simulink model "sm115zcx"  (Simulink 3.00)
settings: Solver=ode45  SolverMode=SingleTasking  StartTime=0.0  StopTime=2.0  RelTol=1e-3  AbsTol=1e-6

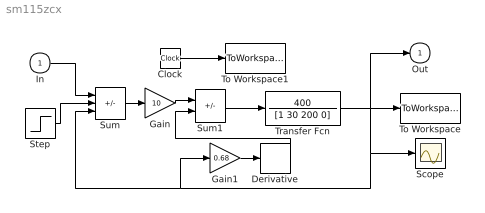
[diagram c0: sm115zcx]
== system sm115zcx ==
  In : Inport  Port=1  PortWidth=-1  SampleTime=-1  DataType=auto
  Clock : Clock
  Derivative : Derivative
  Gain : Gain  Gain=10  SaturateOnIntegerOverflow=on
  Gain1 : Gain  Gain=0.68  SaturateOnIntegerOverflow=on
  Scope : Scope
  Step : Step  Time=0  Before=0  After=1  SampleTime=0
  Sum : Sum  Inputs=++-  SaturateOnIntegerOverflow=on
  Sum1 : Sum  Inputs=+-  SaturateOnIntegerOverflow=on
  To Workspace : ToWorkspace  VariableName=y3  SampleTime=-1  SaveFormat=Matrix
  To Workspace1 : ToWorkspace  VariableName=t3  SampleTime=-1  SaveFormat=Matrix
  Transfer Fcn : TransferFcn  Numerator=400  Denominator=[1 30 200 0]
  Out : Outport  Port=1  InitialOutput=0
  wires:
  Clock/1 -> To Workspace1/1
  Sum/1 -> Gain/1
  Gain/1 -> Sum1/1
  Transfer Fcn/1 -> To Workspace/1, Scope/1, Gain1/1, Sum/3, Out/1
  Derivative/1 -> Sum1/2
  Gain1/1 -> Derivative/1
  Step/1 -> Sum/2
  In/1 -> Sum/1
  Sum1/1 -> Transfer Fcn/1
